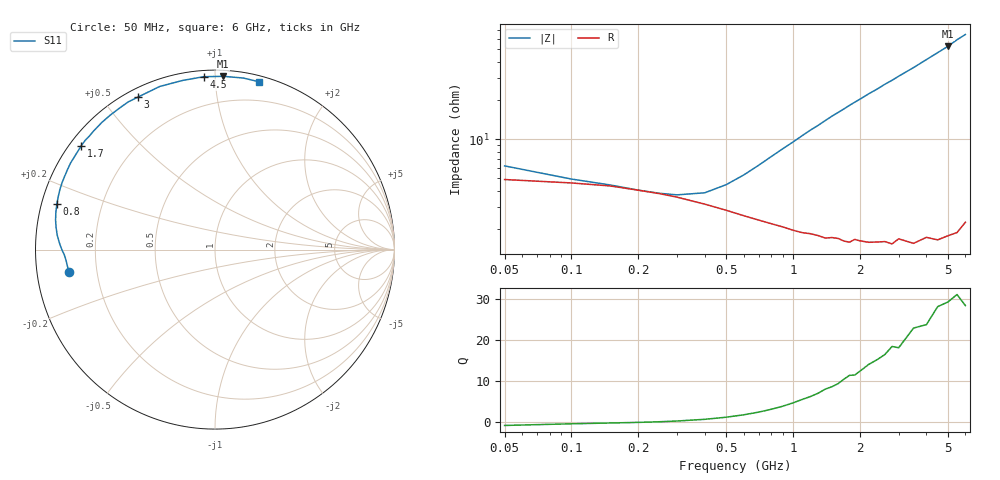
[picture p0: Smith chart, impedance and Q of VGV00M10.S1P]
! Infineon Technologies  Discrete & RF Semiconductors
! BB 831
! Si Tuning Diode in SOD323
! VR =
! S-Parameters:  July  1999
# GHz  S  MA  R  50
!  f  S11
! GHz  MAG  ANG
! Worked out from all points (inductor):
!   34 points, 50 MHz to 6 GHz, reference 50 ohm
!   read as one part to ground: L = 1.5 nH near 800 MHz
!   highest Q = 29.3 at 5 GHz (marker M1), where L = 1.67 nH
!   S11 on the Smith chart (normalised r, x): 50 MHz: 0.10, -0.08; 800 MHz: 0.04, +0.14; 1.7 GHz: 0.03, +0.34; 3 GHz: 0.03, +0.61; 4.5 GHz: 0.03, +0.94; 6 GHz: 0.05, +1.30
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0.05  0.8234 -171.1
0.1  0.8323 -175.9
0.15  0.8403 -178.1
0.2  0.8508 -179.6
0.3  0.8673 177.6
0.4  0.8821 174.9
0.5  0.8939 172.1
0.6  0.9036 169.4
0.7  0.9109 166.7
0.8  0.9168 164.0
1  0.9266 158.9
1.1  0.9302 156.3
1.3  0.9349 151.5
1.4  0.9383 149.0
1.6  0.9402 144.4
1.7  0.9435 142.2
1.8  0.9453 139.9
2.2  0.9485 131.6
2.4  0.9497 127.9
2.6  0.9511 123.9
2.8  0.9545 120.5
3  0.9521 116.8
3.5  0.9596 108.7
4  0.9596 100.8
4.5  0.9653 93.7
5  0.9665 87.3
5.5  0.9688 80.6
6  0.9666 75.3
